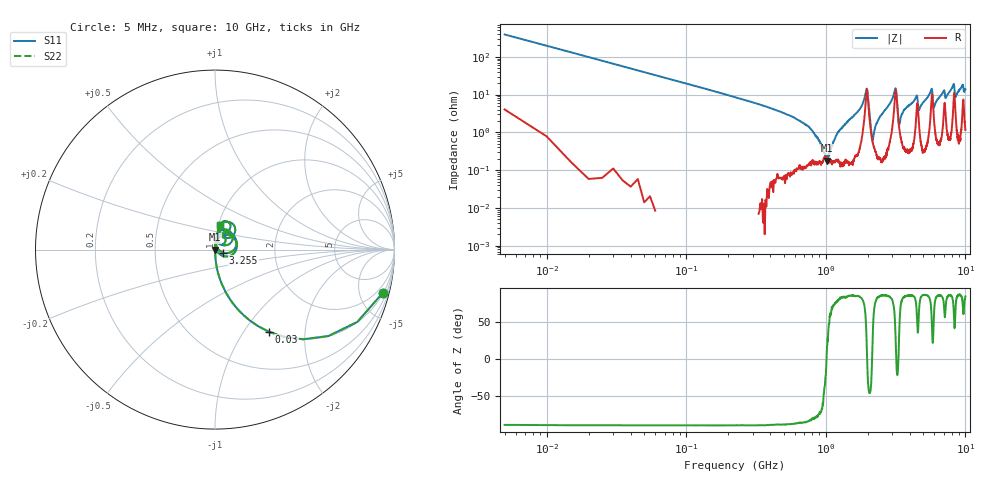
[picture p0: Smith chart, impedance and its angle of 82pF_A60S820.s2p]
! Amotech Co.,Ltd.
! http://www.amotech.co.kr/
! Part Number: A60S820
! These Parameters are Measured in Series Mode Connection
! Operation Temp=25[degC], DC Bias Voltage=0[V]
! Freq. Start=5[MHz] Stop=10[GHz], 2000[Steps]
! Date: Monday, July 13, 2020, 01:44:25
# GHZ S RI R 50.000000
!Freq.(Hz) S11(Real) S11(Imag) S21(Real) S21(Imag) S12(Real) S12(Imag) S22(Real) S22(Imag)
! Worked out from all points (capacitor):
!   2000 points, 5 MHz to 10 GHz, reference 50 ohm
!   read as one part in series: C = 80.5 pF near 55 MHz
!   lowest |Z| = 178 mohm at 1.015 GHz (marker M1)
!   series resonance near 1.013 GHz, so ESL is about 310 pH
!   S11 on the Smith chart (normalised r, x): 5 MHz: 1.08, -7.79; 30 MHz: 1.00, -1.31; 3.255 GHz: 1.09, -0.04; 10 GHz: 1.02, +0.28
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0.005  0.936 -0.2396  0.064 0.2396  0.064 0.2396  0.936 -0.2396
0.03  0.3017 -0.4581  0.6983 0.4581  0.6983 0.4581  0.3017 -0.4581
0.13  0.0219 -0.1473  0.9781 0.1473  0.9781 0.1473  0.0219 -0.1473
0.76  0.00157 -0.0135  0.9984 0.0135  0.9984 0.0135  0.00157 -0.0135
1.015  0.00177 0.000173  0.9982 -0.000173  0.9982 -0.000173  0.00177 0.000173
1.245  0.00181 0.0109  0.9982 -0.0109  0.9982 -0.0109  0.00181 0.0109
1.675  0.00375 0.0337  0.9963 -0.0337  0.9963 -0.0337  0.00375 0.0337
1.965  0.1215 0.0337  0.8785 -0.0337  0.8785 -0.0337  0.1215 0.0337
2.17  0.00535 0.00331  0.9947 -0.00331  0.9947 -0.00331  0.00535 0.00331
2.41  0.00269 0.0236  0.9973 -0.0236  0.9973 -0.0236  0.00269 0.0236
3.13  0.087 0.0895  0.913 -0.0895  0.913 -0.0895  0.087 0.0895
3.255  0.0445 -0.0168  0.9555 0.0168  0.9555 0.0168  0.0445 -0.0168
3.34  0.0149 0.00608  0.9851 -0.00608  0.9851 -0.00608  0.0149 0.00608
4.46  0.0377 0.0808  0.9623 -0.0808  0.9623 -0.0808  0.0377 0.0808
4.645  0.0186 0.0338  0.9814 -0.0338  0.9814 -0.0338  0.0186 0.0338
5.005  0.00703 0.0627  0.993 -0.0627  0.993 -0.0627  0.00703 0.0627
5.72  0.0794 0.1047  0.9206 -0.1047  0.9206 -0.1047  0.0794 0.1047
5.945  0.0243 0.0361  0.9757 -0.0361  0.9757 -0.0361  0.0243 0.0361
6.67  0.015 0.0923  0.985 -0.0923  0.985 -0.0923  0.015 0.0923
8.335  0.108 0.0887  0.892 -0.0887  0.892 -0.0887  0.108 0.0887
8.485  0.0393 0.0715  0.9607 -0.0715  0.9607 -0.0715  0.0393 0.0715
10  0.0301 0.1343  0.9699 -0.1343  0.9699 -0.1343  0.0301 0.1343
